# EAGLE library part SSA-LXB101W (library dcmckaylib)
10 Segment RED LED Lumex
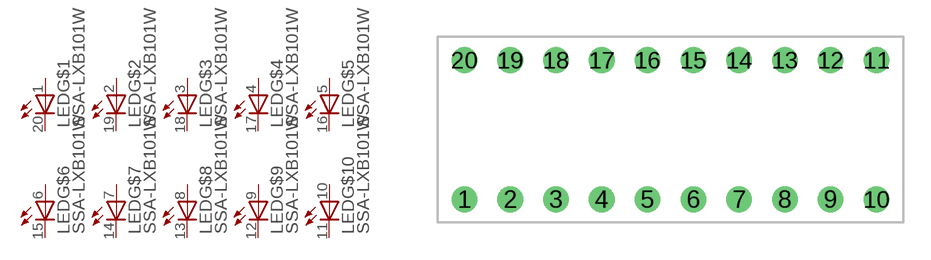
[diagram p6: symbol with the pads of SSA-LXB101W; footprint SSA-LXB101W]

Designator prefix LED; gates G$1=LED G$2=LED G$3=LED G$4=LED G$5=LED G$6=LED G$7=LED G$8=LED G$9=LED G$10=LED

## SSA-LXB101W  [SSA-LXB101W]
1  G$1:ANODE
2  G$2:ANODE
3  G$3:ANODE
4  G$4:ANODE
5  G$5:ANODE
6  G$6:ANODE
7  G$7:ANODE
8  G$8:ANODE
9  G$9:ANODE
10  G$10:ANODE
11  G$10:CATHODE
12  G$9:CATHODE
13  G$8:CATHODE
14  G$7:CATHODE
15  G$6:CATHODE
16  G$5:CATHODE
17  G$4:CATHODE
18  G$3:CATHODE
19  G$2:CATHODE
20  G$1:CATHODE

## Footprint SSA-LXB101W (pad centres in mm)
drill 0.889: 1 -11.254,-3.81; 2 -8.754,-3.81; 3 -6.254,-3.81; 4 -3.754,-3.81; 5 -1.254,-3.81; 6 1.246,-3.81; 7 3.746,-3.81; 8 6.246,-3.81; 9 8.746,-3.81; 10 11.246,-3.81; 11 11.246,3.81; 12 8.746,3.81; 13 6.246,3.81; 14 3.746,3.81; 15 1.246,3.81; 16 -1.254,3.81; 17 -3.754,3.81; 18 -6.254,3.81; 19 -8.754,3.81; 20 -11.254,3.81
